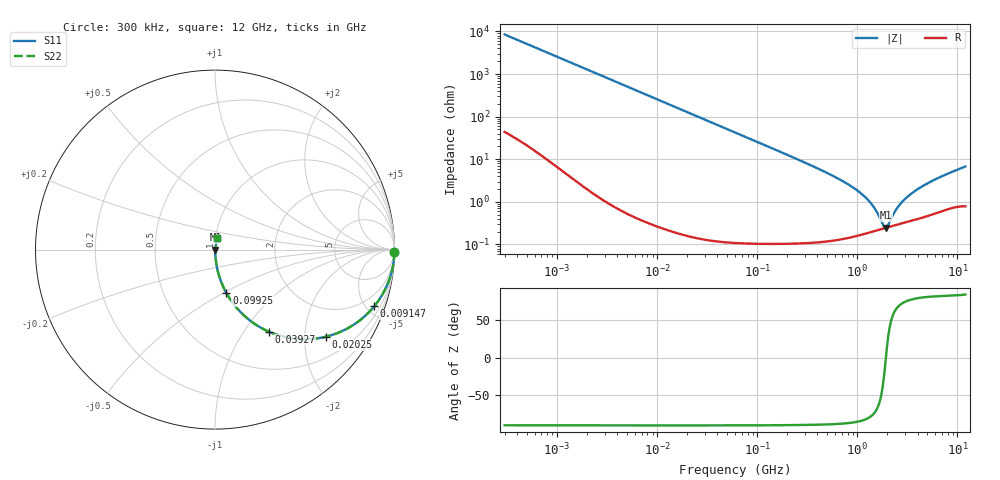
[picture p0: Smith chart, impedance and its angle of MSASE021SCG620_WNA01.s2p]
! MSASE021SCG620_WNA01  S-PARAMETER MODEL  ( Standard Model )
! Model Generated by TAIYO YUDEN Corporation (http://www.ty-top.com)
! Version 1.0
! TAIYO YUDEN Control No. 241126
! Copyright(c) 2024 TAIYO YUDEN CO.,LTD. All Rights Reserved.
! Product Description (link to TY-COMPAS)
! https://ds.yuden.co.jp/TYCOMPAS/or/detail?pn=MSASE021SCG620GWNA01&u=M
! Products Name : Multilayer Ceramic Capacitors
! Characteristics :
!  Capacitance : 62 [pF] , Rated Voltage : 16 [V] , TCC : CG / C0G
!  Case Size : 0.25 x 0.125 / 0.0098 x 0.0049 [mm/inch] , Thickness : 0.125 / 0.0049 [mm/inch]
!  (Conditions: Temperature = 25 [degC] , DC Bias Voltage = 0 [V])
! External Node Assignments :
!  1  o---| |---o  2
! GND o---------o GND
! Frequency Range : 0.3MHz  -  12000MHz  [ 401 STEP ]
# MHZ S RI R 50
! Freq[MHz].  S11 Real  S11 Imag  S21 Real  S21 Imag  S12 Real  S12 Imag  S22 Real  S22 Imag
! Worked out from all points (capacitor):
!   401 points, 300 kHz to 12 GHz, reference 50 ohm
!   read as one part in series: C = 62.3 pF near 316.3 kHz
!   lowest |Z| = 246 mohm at 1.929 GHz (marker M1)
!   series resonance near 1.929 GHz, so ESL is about 110 pH
!   S11 on the Smith chart (normalised r, x): 300 kHz: open; 9.147 MHz: 1.01, -5.61; 20.25 MHz: 1.00, -2.53; 39.27 MHz: 1.00, -1.31; 99.25 MHz: 1.00, -0.52; 12 GHz: 1.02, +0.13
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0.3  0.9998 -0.0117  0.000199 0.0117  0.000199 0.0117  0.9998 -0.0117
1.769972  0.9951 -0.0687  0.00486 0.0687  0.00486 0.0687  0.9951 -0.0687
4.131722  0.9745 -0.157  0.0255 0.157  0.0255 0.157  0.9745 -0.157
9.147146  0.8869 -0.3163  0.1131 0.3163  0.1131 0.3163  0.8869 -0.3163
10.44266  0.8575 -0.3491  0.1425 0.3491  0.1425 0.3491  0.8575 -0.3491
20.2507  0.6158 -0.4858  0.3842 0.4858  0.3842 0.4858  0.6158 -0.4858
27.82928  0.4593 -0.4976  0.5407 0.4976  0.5407 0.4976  0.4593 -0.4976
39.27072  0.2992 -0.457  0.7008 0.457  0.7008 0.457  0.2992 -0.457
60  0.1549 -0.3605  0.8451 0.3605  0.8451 0.3605  0.1549 -0.3605
99.25425  0.0631 -0.2412  0.9369 0.2412  0.9369 0.2412  0.0631 -0.2412
353.9943  0.00592 -0.0693  0.9941 0.0693  0.9941 0.0693  0.00592 -0.0693
704.9044  0.00229 -0.0311  0.9977 0.0311  0.9977 0.0311  0.00229 -0.0311
1076.992  0.00192 -0.016  0.9981 0.016  0.9981 0.016  0.00192 -0.016
1403.667  0.00205 -0.00828  0.998 0.00828  0.998 0.00828  0.00205 -0.00828
1560.575  0.00216 -0.00544  0.9978 0.00544  0.9978 0.00544  0.00216 -0.00544
1829.429  0.00237 -0.00134  0.9976 0.00134  0.9976 0.00134  0.00237 -0.00134
1928.972  0.00245 2.69e-07  0.9975 -2.69e-07  0.9975 -2.69e-07  0.00245 2.69e-07
2088.533  0.00259 0.002  0.9974 -0.002  0.9974 -0.002  0.00259 0.002
2581.562  0.00302 0.00733  0.997 -0.00733  0.997 -0.00733  0.00302 0.00733
3547.679  0.00388 0.0158  0.9961 -0.0158  0.9961 -0.0158  0.00388 0.0158
5868.704  0.00623 0.032  0.9938 -0.032  0.9938 -0.032  0.00623 0.032
12000  0.0122 0.0658  0.9878 -0.0658  0.9878 -0.0658  0.0122 0.0658
